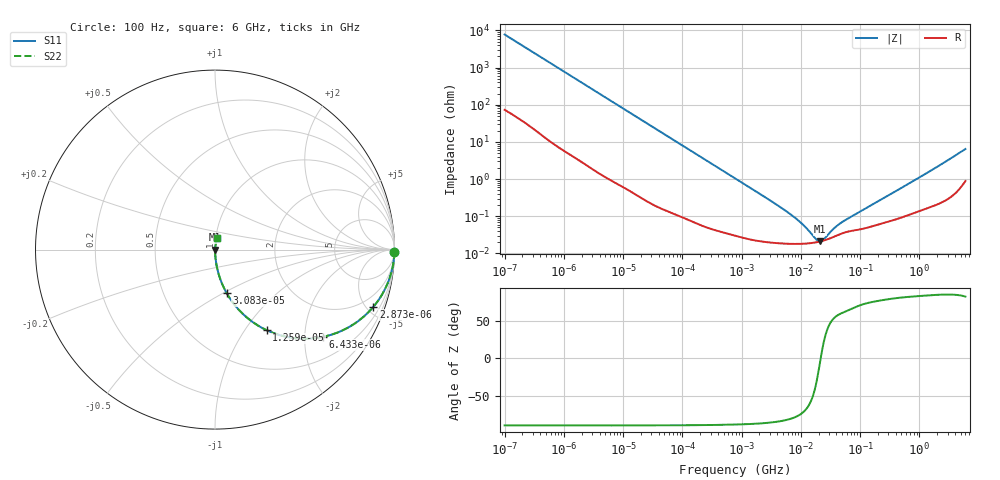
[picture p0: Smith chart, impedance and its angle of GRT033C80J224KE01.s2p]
!Murata Part Number: GRT033C80J224KE01
!These Parameters are Measured in Series Mode Connection
!Data Generated on Jun 19, 2026
!  o--ll--o
!Port1  Port2
!  o------o
!Operation Temp=25[degC], DC Bias Voltage=0[V]
!Freq. Start=100[Hz] Stop=6[GHz] 401[Steps]
# Hz S RI R 50
!Freq.(Hz) S11(Real) S11(Imag) S21(Real) S21(Imag) S12(Real) S12(Imag) S22(Real) S22(Imag)
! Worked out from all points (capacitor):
!   401 points, 100 Hz to 6 GHz, reference 50 ohm
!   read as one part in series: C = 204 nF near 109 Hz
!   lowest |Z| = 21.1 mohm at 21.28 MHz (marker M1)
!   series resonance near 21.68 MHz, so ESL is about 260 pH
!   S11 on the Smith chart (normalised r, x): 100 Hz: open; 2.873 kHz: 1.04, -5.51; 6.433 kHz: 1.02, -2.47; 12.59 kHz: 1.01, -1.26; 30.83 kHz: 1.00, -0.52; 6 GHz: 1.02, +0.13
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100  0.9997 -0.0129  0.000286 0.0129  0.000286 0.0129  0.9997 -0.0129
600  0.9936 -0.0758  0.00636 0.0758  0.00636 0.0758  0.9936 -0.0758
2008  0.9378 -0.2379  0.0622 0.2379  0.0622 0.2379  0.9378 -0.2379
2873  0.8818 -0.3194  0.1182 0.3194  0.1182 0.3194  0.8818 -0.3194
4299  0.771 -0.4166  0.229 0.4166  0.229 0.4166  0.771 -0.4166
6433  0.6029 -0.4857  0.3971 0.4857  0.3971 0.4857  0.6029 -0.4857
12592  0.2873 -0.4486  0.7127 0.4486  0.7127 0.4486  0.2873 -0.4486
19704  0.1429 -0.3461  0.8571 0.3461  0.8571 0.3461  0.1429 -0.3461
30832  0.0648 -0.242  0.9352 0.242  0.9352 0.242  0.0648 -0.242
40335  0.0394 -0.1903  0.9606 0.1903  0.9606 0.1903  0.0394 -0.1903
129199  0.00465 -0.062  0.9954 0.062  0.9954 0.062  0.00465 -0.062
774597  0.000411 -0.0105  0.9996 0.0105  0.9996 0.0105  0.000411 -0.0105
6353432  0.000183 -0.00119  0.9998 0.00119  0.9998 0.00119  0.000183 -0.00119
1.039699e7  0.000182 -0.000612  0.9998 0.000612  0.9998 0.000612  0.000182 -0.000612
1.555665e7  0.000192 -0.000256  0.9998 0.000256  0.9998 0.000256  0.000192 -0.000256
1.86079e7  0.000201 -0.000115  0.9998 0.000115  0.9998 0.000115  0.000201 -0.000115
2.128304e7  0.000211 -1.35e-05  0.9998 1.35e-05  0.9998 1.35e-05  0.000211 -1.35e-05
2.434276e7  0.000223 8.63e-05  0.9998 -8.63e-05  0.9998 -8.63e-05  0.000223 8.63e-05
3.64232e7  0.000282 0.000382  0.9997 -0.000382  0.9997 -0.000382  0.000282 0.000382
4.983056e7  0.000347 0.000609  0.9997 -0.000609  0.9997 -0.000609  0.000347 0.000609
3.124326e8  0.000744 0.0037  0.9993 -0.0037  0.9993 -0.0037  0.000744 0.0037
6e9  0.0128 0.0626  0.9872 -0.0626  0.9872 -0.0626  0.0128 0.0626
